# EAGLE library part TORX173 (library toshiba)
FIBER OPTIC RECEIVING MODULE FOR DIGITAL AUDIO EQUIPMENT, TTL Interface TORX173.pdf
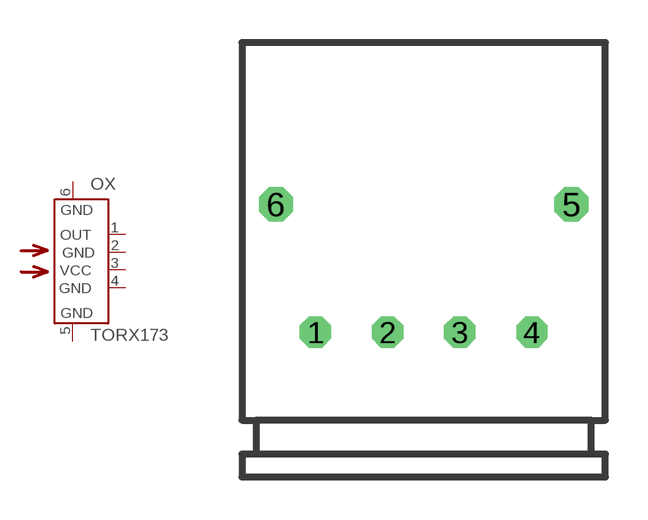
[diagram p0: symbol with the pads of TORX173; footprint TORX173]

Designator prefix OX

## TORX173 (OC_FARNELL: unknown; OC_NEWARK: unknown)  [TORX173]
1  OUT  out
2  GND  pwr
3  VCC  pwr
4  GND  pwr
5  GND  pwr
6  GND  pwr

## Footprint TORX173 (pad centres in mm)
FIBER OPTIC RECEIVING MODULE FOR DIGITAL AUDIO EQUIPMENT; TTL Interface TORX173.pdf
drill 0.6 octagon: 1 -3.81,0; 2 -1.27,0; 3 1.27,0; 4 3.81,0
drill 0.7 octagon: 5 5.2,4.5; 6 -5.2,4.5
